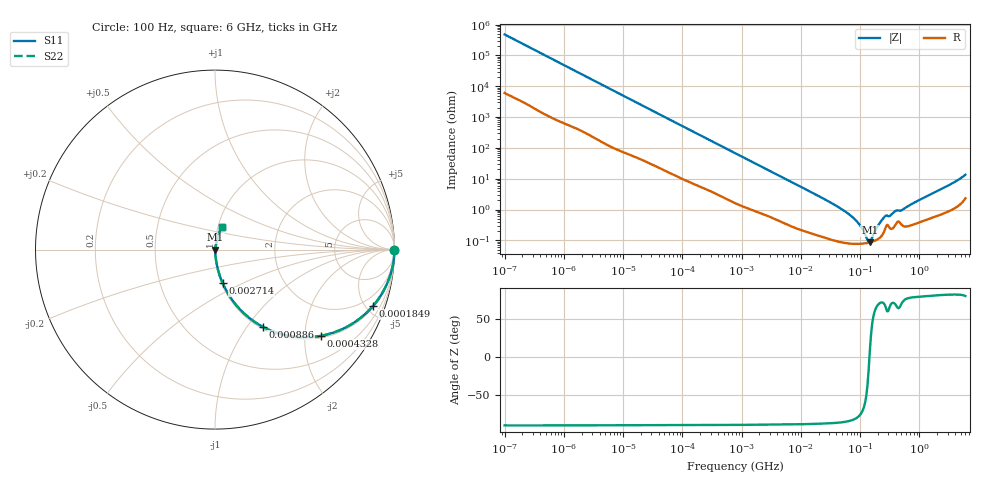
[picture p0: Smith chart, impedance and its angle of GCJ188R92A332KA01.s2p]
!Murata Part Number: GCJ188R92A332KA01
!These Parameters are Measured in Series Mode Connection
!Data Generated on Mar 13, 2026
!  o--ll--o
!Port1  Port2
!  o------o
!Operation Temp=25[degC], DC Bias Voltage=0[V]
!Freq. Start=100[Hz] Stop=6[GHz] 401[Steps]
# Hz S RI R 50
!Freq.(Hz) S11(Real) S11(Imag) S21(Real) S21(Imag) S12(Real) S12(Imag) S22(Real) S22(Imag)
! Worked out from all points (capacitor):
!   401 points, 100 Hz to 6 GHz, reference 50 ohm
!   read as one part in series: C = 3.32 nF near 109 Hz
!   lowest |Z| = 86.3 mohm at 145.9 MHz (marker M1)
!   series resonance near 144.1 MHz, so ESL is about 370 pH
!   S11 on the Smith chart (normalised r, x): 100 Hz: open; 184.9 kHz: 1.12, -5.55; 432.8 kHz: 1.06, -2.40; 886 kHz: 1.03, -1.18; 2.714 MHz: 1.01, -0.39; 6 GHz: 1.05, +0.27
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100  1 -0.000209  2.7e-06 0.000209  2.7e-06 0.000209  1 -0.000209
2008  0.9999 -0.0041  7.56e-05 0.0041  7.56e-05 0.0041  0.9999 -0.0041
40335  0.9922 -0.0792  0.00776 0.0792  0.00776 0.0792  0.9922 -0.0792
184852  0.8801 -0.3144  0.1199 0.3144  0.1199 0.3144  0.8801 -0.3144
432798  0.5888 -0.4806  0.4112 0.4806  0.4112 0.4806  0.5888 -0.4806
774597  0.3181 -0.454  0.6819 0.454  0.6819 0.454  0.3181 -0.454
885955  0.2649 -0.4293  0.7351 0.4293  0.7351 0.4293  0.2649 -0.4293
1449809  0.1239 -0.3162  0.8761 0.3162  0.8761 0.3162  0.1239 -0.3162
2713602  0.0429 -0.1874  0.9571 0.1874  0.9571 0.1874  0.0429 -0.1874
1.555665e7  0.00286 -0.035  0.9971 0.035  0.9971 0.035  0.00286 -0.035
4.165952e7  0.00107 -0.0124  0.9989 0.0124  0.9989 0.0124  0.00107 -0.0124
7.129496e7  0.000811 -0.00603  0.9992 0.00603  0.9992 0.00603  0.000811 -0.00603
9.753859e7  0.000777 -0.00318  0.9992 0.00318  0.9992 0.00318  0.000777 -0.00318
1.334425e8  0.000824 -0.000613  0.9992 0.000613  0.9992 0.000613  0.000824 -0.000613
1.459435e8  0.000856 0.000106  0.9991 -0.000106  0.9991 -0.000106  0.000856 0.000106
2.388273e8  0.00153 0.00453  0.9985 -0.00453  0.9985 -0.00453  0.00153 0.00453
2.61201e8  0.00218 0.00548  0.9978 -0.00548  0.9978 -0.00548  0.00218 0.00548
3.124326e8  0.00262 0.00544  0.9974 -0.00544  0.9974 -0.00544  0.00262 0.00544
3.908258e8  0.00314 0.00821  0.9969 -0.00821  0.9969 -0.00821  0.00314 0.00821
5.112761e8  0.00318 0.00908  0.9968 -0.00908  0.9968 -0.00908  0.00318 0.00908
2.142435e9  0.00812 0.0409  0.9919 -0.0409  0.9919 -0.0409  0.00812 0.0409
6e9  0.039 0.1249  0.961 -0.1249  0.961 -0.1249  0.039 0.1249
